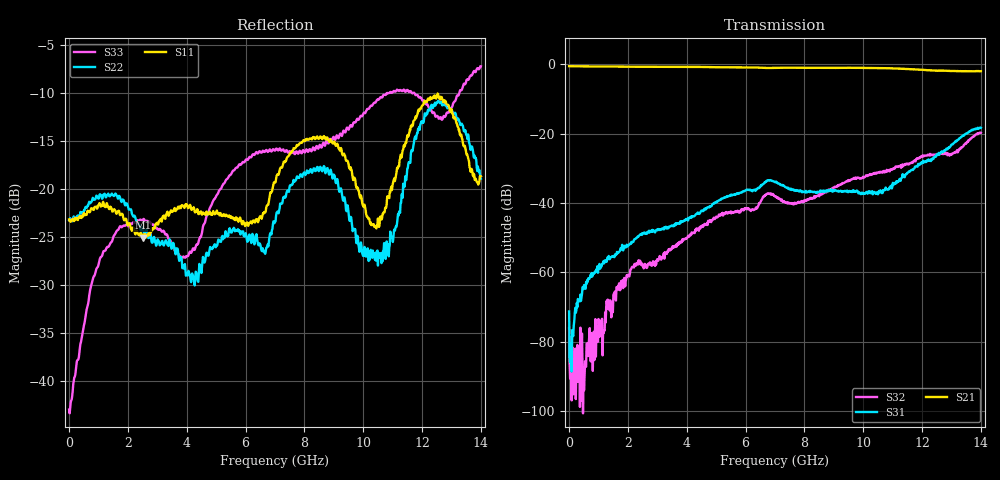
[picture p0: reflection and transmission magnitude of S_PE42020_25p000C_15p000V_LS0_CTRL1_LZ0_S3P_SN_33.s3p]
! Device ID: PE42020
! File Path: z:\PE42020\sparam_retest1\25p000C\3p000\LS_CTRL1_LZ0\PE42020_25p000C_3p000V_3p000V_0p000V_LS_CTRL1_LZ0_S3P_SN_33__2_3.s3p
! Serial: 33
! Lot:
! Temp: 25.000C
! VDD: 15.000
! VSS: -15.000
! Control_Hi: 3.000
! Control_Lo: 0.000
! Logic State: LS_CTRL1_LZ0
! Port 1: RFC
! Port 3: RF2
! Port 4:
! ThroughPath:1-3
! IDD: -0.0020676223
! ISS: 0
! Comment:
#  Hz  S  RI  R  50
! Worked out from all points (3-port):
!   801 points, 300 kHz to 14 GHz, reference 50 ohm
!   strongest paths, dB at 300 kHz, 3.5 GHz, 7 GHz, 10.5 GHz, 14 GHz:
!     S21: -0.6, -0.8, -1.1, -1.2, -2.0
!     S31: -71.2, -46.4, -34.0, -37.5, -18.3
!     S32: -76.0, -53.1, -38.1, -31.2, -19.8
!   lowest |S11| = -25.0 dB at 2.503 GHz (marker M1), VSWR 1.12, Z = 54.5 - j3.77 ohm
!   |S11| at or under -10 dB: start of sweep to end of sweep
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300000  0.0697 0.00369  0.9351 0.00324  0.000875 0.000725
        0.9336 0.00311  0.0689 0.00344  -0.000346 -0.000212
        0.000224 -0.00016  -0.000147 -6.07e-05  0.00681 -0.00211
8.78e7  0.0693 -0.0069  0.9319 -0.0232  -2.96e-05 3.19e-05
        0.933 -0.0221  0.0695 -0.00564  1.09e-05 -3.07e-05
        2.07e-05 3.14e-05  -1.06e-07 1.44e-05  0.00749 -0.00293
6.828e8  0.0628 -0.0445  0.9109 -0.1596  2.6e-05 0.000844
         0.9125 -0.1597  0.0721 -0.0472  -4.12e-05 4.06e-05
         4.89e-05 0.000804  -9.35e-05 6.88e-05  0.016 -0.0229
2.5028e9  0.0442 -0.0345  0.7458 -0.5286  -3.63e-05 0.00361
          0.7457 -0.5302  0.051 -0.0377  -0.00079 0.0011
          0.000168 0.00366  -0.000723 0.000989  0.0617 -0.0317
3.9903e9  0.0665 -0.051  0.5076 -0.7594  -1.68e-05 0.00585
          0.5084 -0.7604  0.0338 -0.0132  -0.00237 0.00214
          -3.39e-05 0.0058  -0.00208 0.0023  0.022 -0.039
7.0003e9  0.0574 -0.092  -0.1245 -0.8745  0.0161 0.012
          -0.1262 -0.8746  0.0596 -0.0328  0.00656 0.0105
          0.0161 0.0118  0.00663 0.0105  -0.0197 -0.1579
8.7153e9  0.0844 -0.1618  -0.4753 -0.7423  0.0128 0.0072
          -0.4774 -0.7424  0.1039 -0.0627  0.00735 0.0126
          0.0129 0.00715  0.00747 0.0127  -0.1205 -0.1219
1.04828e10  -0.0279 -0.0593  -0.7561 -0.4468  0.011 0.00953
            -0.7559 -0.4449  -0.0288 -0.0384  0.0238 0.0135
            0.0106 0.00939  0.0239 0.013  -0.2927 -0.0246
1.23728e10  -0.1288 -0.2705  -0.8101 -0.0334  0.0283 0.036
            -0.8091 -0.0322  0.0619 -0.2584  0.0476 -0.00263
            0.0265 0.0346  0.0488 -0.000502  -0.1783 0.1772
1.40003e10  0.1129 -0.0303  -0.7486 0.2493  0.1186 0.0258
            -0.7481 0.2542  0.1089 -0.0326  0.096 -0.0391
            0.1182 0.0267  0.0938 -0.0417  0.3058 0.3132
